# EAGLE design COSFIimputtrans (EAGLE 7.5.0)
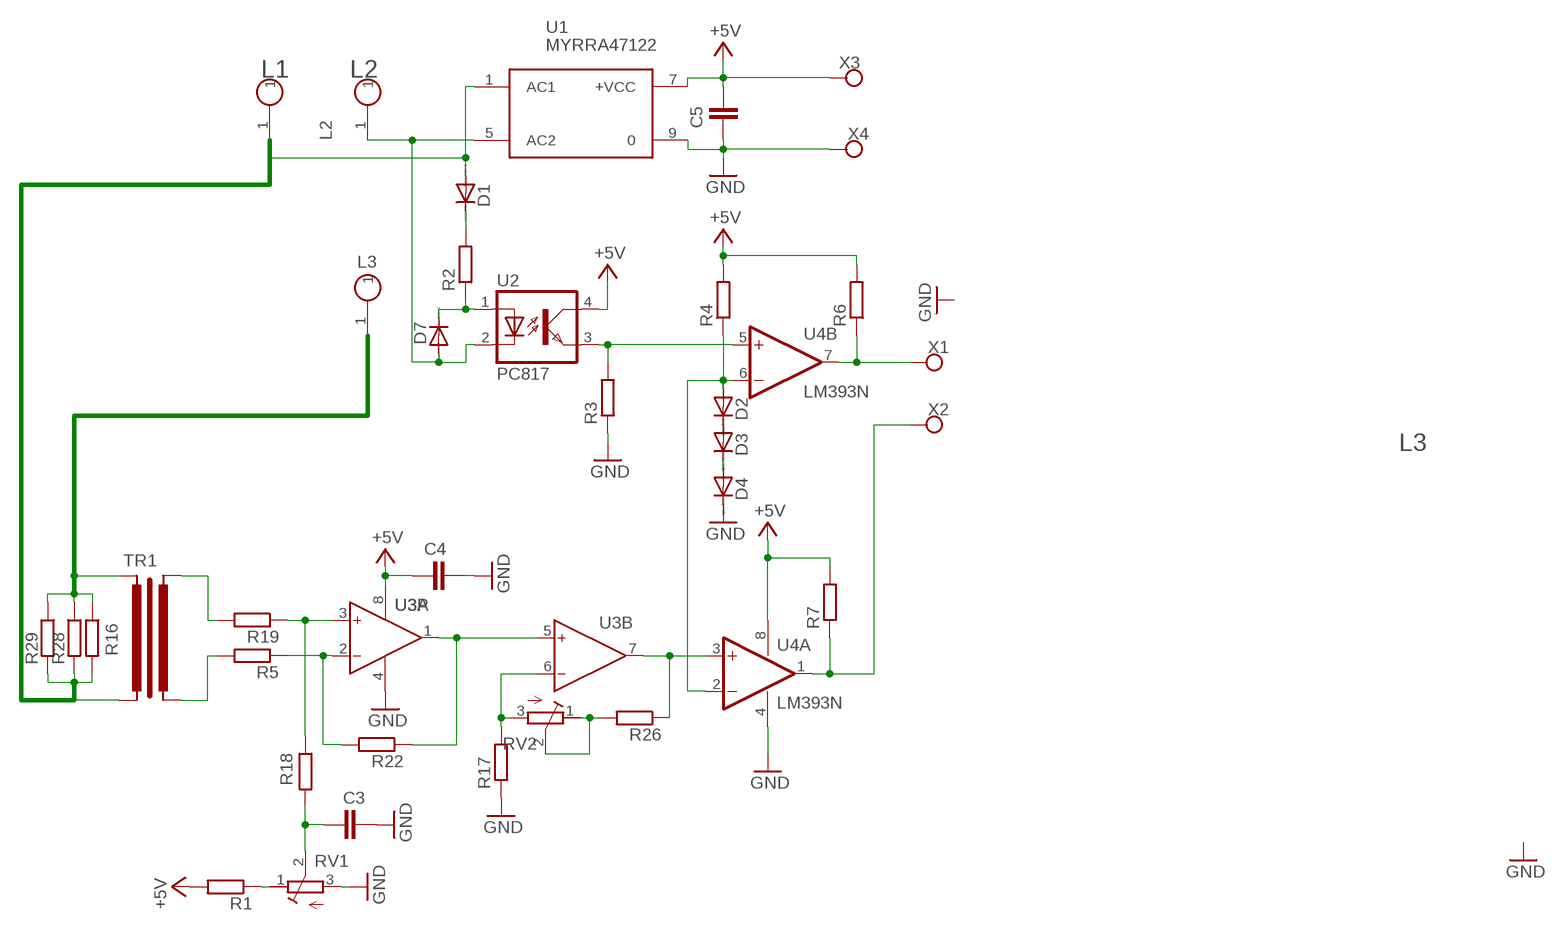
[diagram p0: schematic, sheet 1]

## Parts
C3  C-EUC1206  [C1206]
C4  C-EUC1206  [C1206]
C5  C-EUC1206  [C1206]
D1  1N4004  [DO41-10]
D2  1N4148DO35-7  [DO35-7]
D3  1N4148DO35-7  [DO35-7]
D4  1N4148DO35-7  [DO35-7]
D7  1N4004  [DO41-10]
L1  CONNHOLE  [CONNHOLE4]
L2  CONNHOLE  [CONNHOLE4]
L3  CONNHOLE  [CONNHOLE4]
R1  R-EU_0204/7  [0204/7]
R2  R-EU_0617/22  [0617/22]
R3  R-EU_0204/7  [0204/7]
R4  R-EU_0204/7  [0204/7]
R5  R-EU_0204/7  [0204/7]
R6  R-EU_0204/7  [0204/7]
R7  R-EU_0204/7  [0204/7]
R16  SHUNT40MM  [SHUNT40MM]
R17  R-EU_0204/7  [0204/7]
R18  R-EU_0204/7  [0204/7]
R19  R-EU_0204/7  [0204/7]
R22  R-EU_0204/7  [0204/7]
R26  R-EU_0204/7  [0204/7]
R28  SHUNT40MM  [SHUNT40MM]
R29  SHUNT40MM  [SHUNT40MM]
RV1  R-TRIMM-3386-F  [R-TRIMM-3386F]
RV2  R-TRIMM-3386-F  [R-TRIMM-3386F]
TR1  TRAFOTOR55  [TRAFOTOR55]
U1  MYRRA47122  [MYRRA47122]
U2  PC817  [DIL04]
U3  AD8042N  [DIL08]
U4  LM393N  [DIL08]
X1  CONNWIRE  [CONNWIRE]
X2  CONNWIRE  [CONNWIRE]
X3  CONNWIRE  [CONNWIRE]
X4  CONNWIRE  [CONNWIRE]

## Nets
+5V: C4.1 C5.2 R1.2 R4.2 R6.2 R7.2 U1.7(+VCC) U2.4(COL) U3.8(P:V+) U4.8(P:V+) X3.P$1
GND: C3.1 C4.2 C5.1 D4.C R3.1 R17.1 RV1.3(E) U1.9 U3.4(P:V-) U4.4(P:V-) X4.P$1
N$1: R26.2 RV2.1(A) RV2.2(S)
N$2: R26.1 U3.7(B:OUT) U4.3(A:+IN)
N$3: D7.C R2.1 U2.1(A)
N$4: D2.C D3.A
N$5: D7.A L2.1 U1.5(AC2) U2.2(C)
N$7: R17.2 RV2.3(E) U3.6(B:IN-)
N$8: D3.C D4.A
N$9: R22.1 U3.1(A:OUT) U3.5(B:IN+)
N$10: D1.C R2.2
N$11: R19.2 TR1.4
N$12: R5.1 R22.2 U3.2(A:IN-)
N$13: R3.2 U2.3(EMIT) U4.5(B:+IN)
N$14: R1.1 RV1.1(A)
N$15: R18.1 R19.1 U3.3(A:IN+)
N$16: D2.A R4.1 U4.2(A:-IN) U4.6(B:-IN)
N$17: R7.1 U4.1(A:OUT) X2.P$1
N$18: R6.1 U4.7(B:OUT) X1.P$1
N$20: C3.2 R18.2 RV1.2(S)
N$21: R5.2 TR1.3
N$22: L3.1 R16.1 R28.1 R29.1 TR1.1
N$23: D1.A L1.1 R16.2 R28.2 R29.2 TR1.2 U1.1(AC1)

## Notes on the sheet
- L1 | L2
- L3

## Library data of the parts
C3-C5 = rcl:C-EU: CAPACITOR, European symbol
D1 D7 = diode:1N4004: DIODE
D2-D4 = diode:1N4148: DIODE
L1-L3 = connholes:CONNHOLE
R1-R7 R17-R19 R22 R26 = rcl:R-EU_: RESISTOR, European symbol
R16 R28 R29 = resistor-shunt:SHUNT40MM
RV1 RV2 = rcl:R-TRIMM-3386-F
TR1 = trafo:TRAFOTOR55
U1 = acdc:MYRRA47122: AC-DC CONVERTER 5V 550mA
U2 = optocoupler:PC817: SHARP OPTO COUPLER; MPN: PC817X4J000F; OC_FARNELL: 9707727; OC_NEWARK: 97K7059
U3 = analog-devices:AD8042: Dual 160 MHz Rail-to-Rail Amplifier Source: http://www.analog.com/static/imported-files/data_sheets/AD8042.pdf; MF: ANALOG DEVICES; MPN: AD8042AN; OC_FARNELL: 1540543; OC_NEWARK: 52F8033
U4 = linear:LM393: COMPARATOR
X1-X4 = connholes:CONNWIRE

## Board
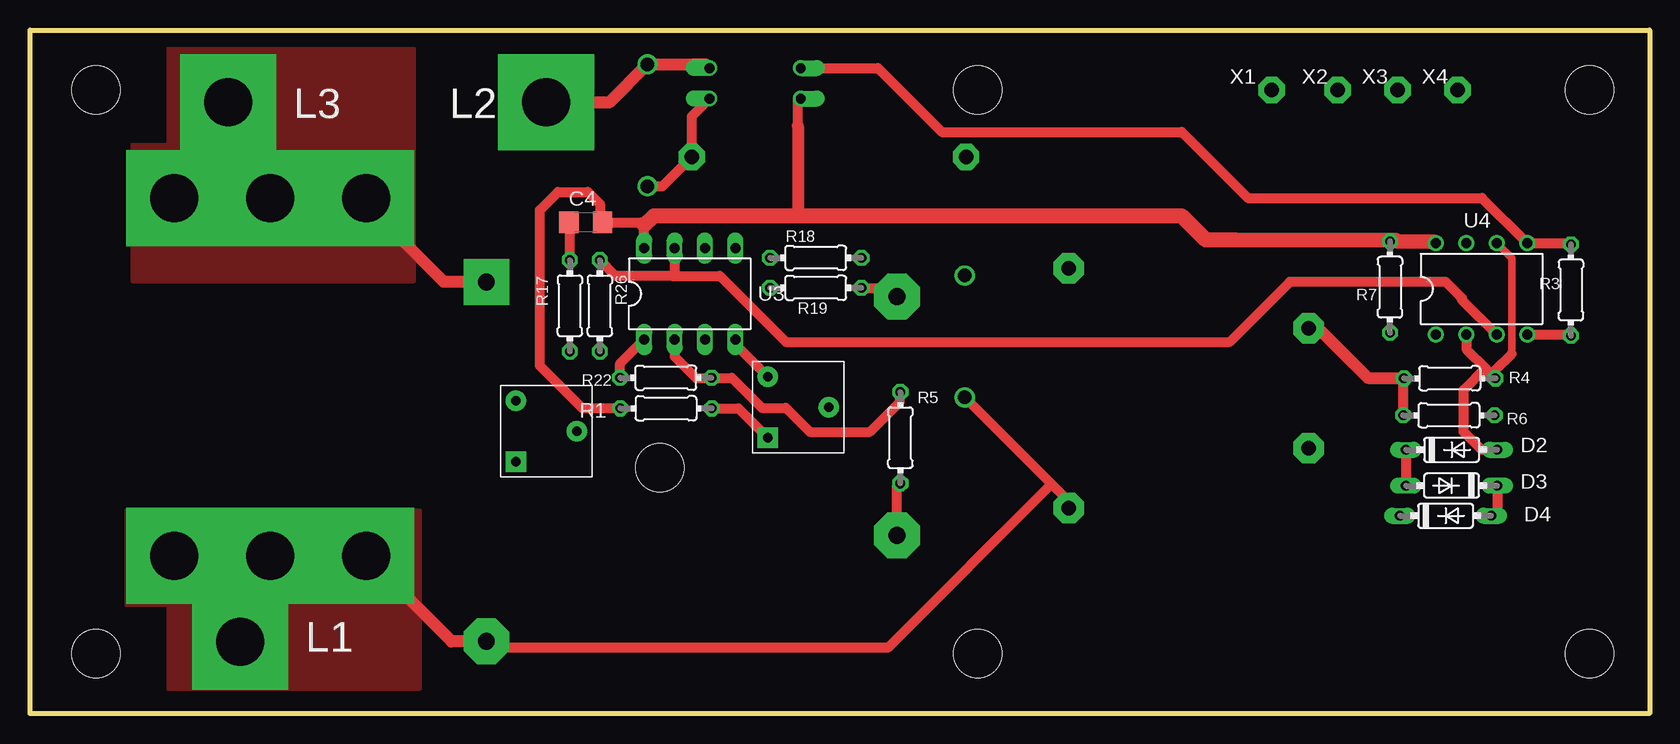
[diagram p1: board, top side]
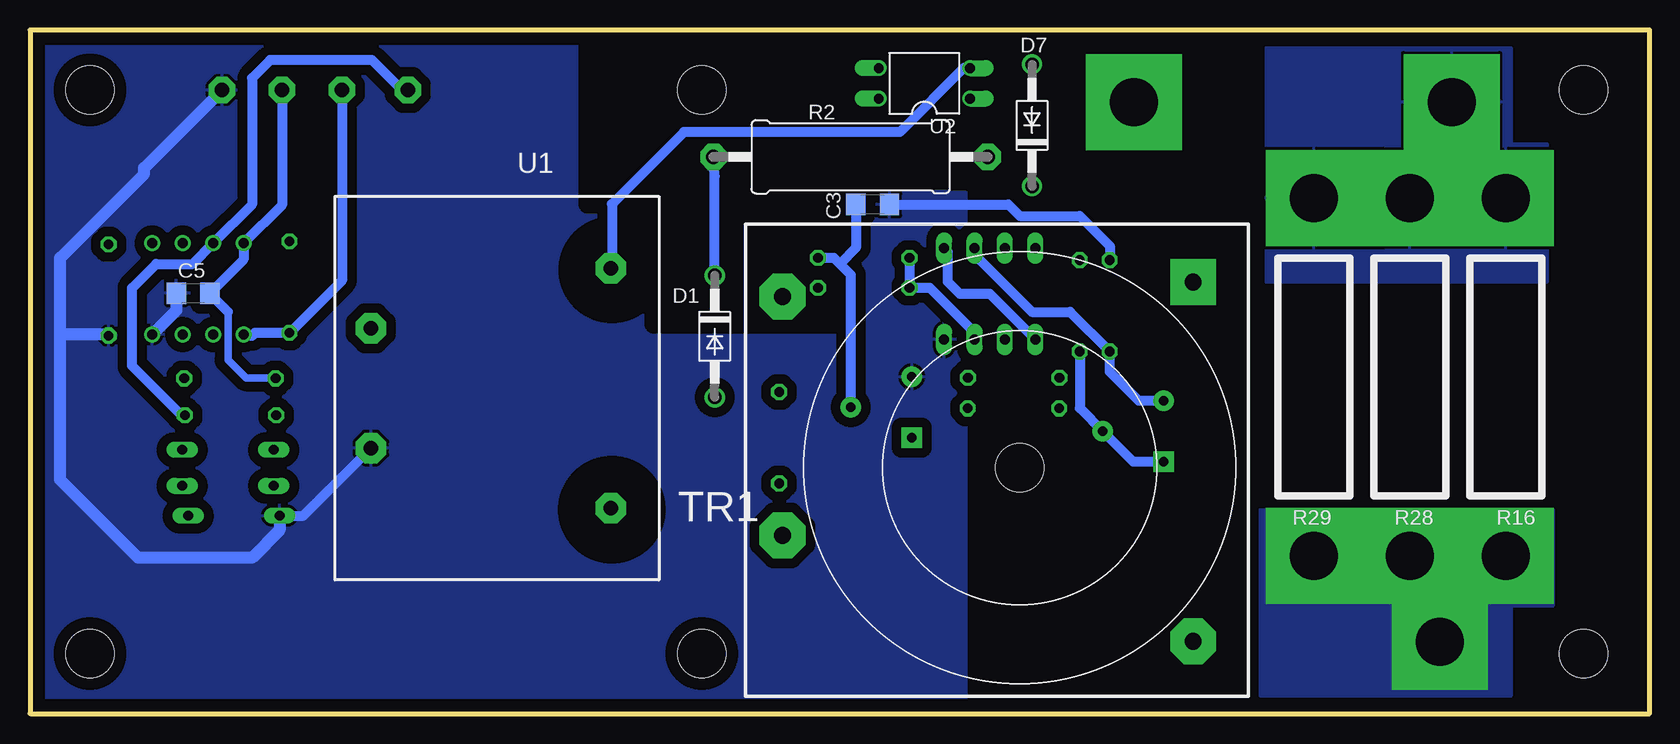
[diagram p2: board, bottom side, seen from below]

Size 135 x 57 mm. Coordinates in mm from the lower left corner, seen from the top.
Outline: 0,0 0,57 135,57 135,0 0,0
Copper layers (1*16): Top 0.035mm / dielectric 1.5mm / Bottom 0.035mm
Design rules "default": minimum track width 10mil, minimum drill 24mil, track to track 8mil, track to pad 8mil, pad to pad 8mil, via to via 8mil, smd to smd 8mil, copper to edge 40mil, drill to drill 8mil, minimum pad ring 10mil, minimum via ring 8mil, stop-mask expansion 4mil, vias tented up to drill 0mil, thermal gap 10mil
Holes 4 mm at 5.5,5 5.5,52 130,52 130,5 79,52 79,5
bRestrict: area 83,33.5 to 90,40.5; area 83,13.5 to 90,20.5; area 58.5,44.5 to 70.5,56; area 71,42.5 to 88.5,56; area 79.5,35.5 to 82.5,41.5; area 67.5,32.5 to 83,44

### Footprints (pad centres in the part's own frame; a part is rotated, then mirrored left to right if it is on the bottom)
C1206 = smd 1.6 x 1.8: 1 -1.4,0; 2 1.4,0
DO41-10 = drill 1.118: A 5.08,0; C -5.08,0
DO35-7 = drill 0.813 long: A 3.81,0; C -3.81,0
CONNHOLE4 = drill 4 pad 8 square: 1 0,0
0204/7 = drill 0.813 octagon: 1 -3.81,0; 2 3.81,0
0617/22 = drill 1.2 pad 2.184 octagon: 1 -11.43,0; 2 11.43,0
SHUNT40MM = drill 4 pad 8 square: 1 0,0; 2 29.84,0
R-TRIMM-3386F = drill 0.8 pad 1.676 square: 1 0,0 | drill 0.8 pad 1.676: 2 5.08,2.54; 3 0,5.08
TRAFOTOR55 = drill 1.4 pad 3.81 square: 1 -14.46,-15.48 | drill 1.4 pad 3.81 octagon: 2 -14.46,14.48; 3 19.77,5.65; 4 19.77,-14.27 | hole 4: 0,0
MYRRA47122 = drill 1.2 pad 2.54 octagon: 1 0,0; 5 20,0; 7 15,20; 9 5,20
DIL04 = drill 0.813 offset: 1 -1.27,-3.81; 2 1.27,-3.81; 3 1.27,3.81; 4 -1.27,3.81
DIL08 = drill 0.813 long: 1 -3.81,-3.81; 2 -1.27,-3.81; 3 1.27,-3.81; 4 3.81,-3.81; 5 3.81,3.81; 6 1.27,3.81; 7 -1.27,3.81; 8 -3.81,3.81
DIL08' = drill 0.813 pad 1.27: 1 -3.81,-3.81; 2 -1.27,-3.81; 3 1.27,-3.81; 4 3.81,-3.81; 5 3.81,3.81; 6 1.27,3.81; 7 -1.27,3.81; 8 -3.81,3.81
CONNWIRE = drill 1.2 pad 2.184 octagon: P$1 0,0

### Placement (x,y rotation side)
C3  64.76,42.45 180 bottom
C4  46.32,40.95 180 top
C5  121.4,35.05 0 bottom
D1  77.92,31.45 270 bottom
D2  118.5,22 0 top
D3  118.5,19 180 top
D4  118,16.5 0 top
D7  51.47,49.05 90 bottom
L1  17.5,6 0 top
L2  43,51 0 top
L3  16.5,51 0 top
R1  53.02,25.45 180 top
R2  66.6,46.42 180 bottom
R3  128.45,35.32 90 top
R4  118.34,27.95 180 top
R5  72.55,23 270 top
R6  118.28,24.87 180 top
R7  113.37,35.56 90 top
R16  12,43 270 bottom
R17  45,34 270 top
R18  65.5,38 0 top
R19  65.5,35.5 0 top
R22  53,28 0 top
R26  47.5,34 270 top
R28  20,43 270 bottom
R29  28,43 270 bottom
RV1  61.5,23 0 top
RV2  40.5,21 0 top
TR1  52.5,20.5 180 bottom
U1  86.58,17.13 90 bottom
U2  60.45,52.55 90 bottom
U3  55,35 0 top
U4  LM393N  [DIL08']  121,35.41 0 top
X1  103.5,52 0 top
X2  109,52 0 top
X3  114,52 0 top
X4  119,52 0 top

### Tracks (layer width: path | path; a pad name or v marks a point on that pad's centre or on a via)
+5V
  Top 0.813: U3.8 51.19,40.69 50.93,40.95 C4.1 47.5,41.17 47.5,42.5 46.5,43.5 44,43.5 42.5,42 42.5,29 46.05,25.45 R1.2 | 64,49 64,51.02 U2.4 | R7.2 114,39.37 | 117.04,39.37 U4.8 | R6.2 114.47,27.89 R4.2
  Top 1.016: U1.7 107.37,32.13 111.5,28 114.48,28 R4.2 | 64,41.5 64.5,41.5 64,42 64,49 | 113.87,39.5 114,39.37
  Top 1.2: 114,39.37 117.04,39.37 | 100.5,39.5 113.87,39.5
  Top 1.27: 100.5,39.5 98,39.5 96,41.5 64,41.5 52,41.5 51.19,40.69
  Bottom 0.61: 118.5,33.5 118.5,29.5 117,28 114.58,28 R4.2
  Bottom 0.813: X3.P$1 114,42.41 U4.8 117.19,37.86 C5.2 120,35 118.5,33.5
GND
  Top 0.813: R17.1 45,40.87 C4.2 | U4.4 128.36,31.6 R3.1 | U3.4 58.81,30.77 RV1.3
  Bottom 0.813: C3.1 53.45,42.45 52.5,41.5 47.5,41.5 45,39 R17.1 | D4.C 112.21,16.5 U1.9
  Bottom 1.016: C5.1 122.8,33.61 U4.4 | R3.1 128.36,31.6 132.4,31.6 132.5,31.5 | D4.C 114.19,15.31 116.5,13 126,13 132.5,19.5 132.5,31.5 | 132.5,31.5 132.5,38 125.5,45 125.5,45.5 X4.P$1
  pour Bottom (isolate 0.813): 58.5,55.5 58.5,43.5 57.5,43.5 57,43.5 57,1 134,1 134,56.5 58.5,56.5 58.5,55.5
N$1
  Bottom 0.813: R26.2 47.5,25.46 RV2.2 43.04,21 RV2.1
N$2
  Top 0.813: U3.7 53.73,36.73 53.5,36.5 | 53.5,36.5 57.5,36.5 63,31 100,31 105,36 118,36 119.37,34.63 119.37,34.5 U4.3 | 53.5,36.5 48.81,36.5 R26.1
N$3
  Top 0.813: D7.C 52.72,43.97 R2.1 55.17,49.81 U2.1
N$4
  Top 0.813: D2.C D3.A
N$5
  Top 1.016: L2.1 48.34,51 D7.A 56.33,54.13 U2.2
  Bottom 0.813: U2.2 57.18,53.82 62.5,48.5 80.5,48.5 86.5,42.5 86.5,37.21 U1.5
N$6
  pour Top (no thermals): 12,17 22.5,17 22.5,2 12,2
  pour Bottom (no thermals): 12,17 22.5,17 22.5,1.5 12,1.5
N$7
  Bottom 0.813: RV2.3 42.58,26.08 45,28.5 R17.2 48.31,33.5 51.5,33.5 56.27,38.27 U3.6
N$8
  Top 0.813: D3.C 122.31,17 D4.A
N$9
  Top 0.813: R22.1 49.19,29.19 U3.1
  Bottom 0.813: U3.1 55,35 57.5,35 58.5,36 58.5,38.5 U3.5
N$10
  Bottom 0.813: D1.C 77.92,44.81 R2.2
N$11
  Top 0.813: R19.2 71.54,35.5 TR1.4
N$12
  Top 0.813: U3.2 53.73,29.77 55.5,28 R22.2 58.5,28 61,25.5 63,25.5 65,23.5 70,23.5 72.5,26 72.5,26.76 R5.1
N$13
  Top 0.813: U2.3 70.68,53.82 76,48.5 96,48.5 101.5,43 121.03,43 U4.5 128.36,39.22 R3.2
N$14
  Top 0.813: R1.1 59.05,25.45 RV1.1
N$15
  Bottom 0.813: U3.3 56.27,31.77 60,35.5 R19.1 R18.1
N$16
  Top 0.61: 123.5,30 123.5,37.99 U4.6
  Top 0.813: U4.2 119.73,30.37 121.3,28.8 | 121.3,28.8 R4.1 122.15,28.65 123.5,30 | D2.A 121,22 119.5,23.5 119.5,27 121.3,28.8
N$17
  Bottom 0.813: X2.P$1 109,36.12 R7.1 116.25,31.75 116.5,31.5 117.09,31.5 U4.1
N$18
  Bottom 0.813: R6.1 122.37,24.87 126.5,29 126.5,35.5 124.5,37.5 121.45,37.5 U4.7 116.5,42.45 116.5,53 115,54.5 106.5,54.5 104,52 X1.P$1
N$19
  pour Top (no thermals): 12,55 22,55 22,36 12,36
  pour Bottom (no thermals): 12,55 22,55 22,36 12,36
N$20
  Bottom 0.813: RV1.2 66.58,36.58 67.5,37.5 | 67.5,37.5 68,38 R18.2 | C3.2 66.16,38.84 67.5,37.5
N$21
  Top 0.813: TR1.3 72.27,18.91 R5.2
N$22
  Top 1.016: TR1.1 34.52,35.98 27.5,43 R29.1
  pour Top (isolate 0.254, no thermals): 8.5,47.5 11.5,47.5 11.5,55.5 32,55.5 32,36 8.5,36
  pour Bottom (isolate 0.254): 11.5,55.5 32,55.5 32,36 8.5,36 8.5,47.5 11.5,47.5
N$23
  Top 0.813: 37.5,6.02 38.02,5.5 71.5,5.5 85.15,19.14 | U1.1 86.58,17.71 85.15,19.14 | 85.15,19.14 D1.A
  Top 1.016: TR1.2 37.5,6.02 35.14,6.02 R29.2
  pour Top (isolate 0.254, no thermals): 8,17 32.5,17 32.5,2 11.5,2 11.5,9 8,9 8,9.5
  pour Bottom (isolate 0.254, no thermals): 8,17 32.5,17 32.5,1.5 11.5,1.5 11.5,9 8,9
